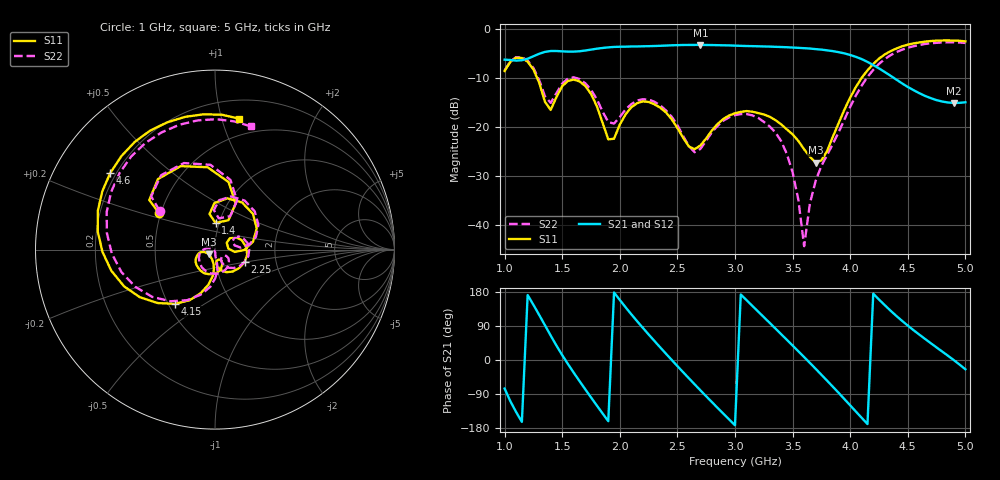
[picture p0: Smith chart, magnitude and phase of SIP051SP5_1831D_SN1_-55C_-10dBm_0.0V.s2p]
# GHz  S  dB  R  50
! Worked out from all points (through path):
!   81 points, 1 GHz to 5 GHz, reference 50 ohm
!   highest |S21| = -3.30 dB at 2.7 GHz (marker M1); lowest = -15.1 dB at 4.9 GHz (marker M2)
!   lowest |S11| = -27.3 dB at 3.7 GHz (marker M3), VSWR 1.09, Z = 46.5 - j2.31 ohm
!   |S11| at or under -10 dB: 1.281 GHz to 4.1 GHz (2.819 GHz wide, 105 % of centre)
!   |S22| runs from -44.3 to -2.8 dB; largest |S21 - S12| = 0.0027
!   S11 on the Smith chart (normalised r, x): 1 GHz: 0.49, +0.23; 1.4 GHz: 0.96, +0.29; 2.25 GHz: 1.38, -0.20; 4.15 GHz: 0.54, -0.38; 4.6 GHz: 0.18, +0.32; 5 GHz: 0.35, +1.14
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1  -8.63 147.1  -6.31 -75.4  -6.31 -75.3  -8.48 144.9
1.2  -6.73 95.1  -6.13 171.4  -6.13 171.4  -6.50 93.1
1.4  -16.57 88.7  -4.55 64.5  -4.56 64.4  -15.12 83.1
1.55  -10.64 76.5  -4.68 -10.8  -4.68 -10.7  -10.17 73.0
1.7  -11.67 27.0  -4.46 -77.3  -4.47 -77.3  -11.12 29.6
1.95  -22.42 30.2  -3.72 178.1  -3.74 178.2  -19.34 25.4
2.1  -16.01 19.3  -3.63 120.6  -3.64 120.6  -15.38 21.1
2.25  -14.94 -23.1  -3.57 67.4  -3.57 67.4  -14.45 -11.0
2.35  -16.08 -51.2  -3.49 33.5  -3.48 33.5  -15.62 -33.5
2.5  -20.24 -82.4  -3.37 -16.1  -3.36 -16.0  -19.66 -59.8
2.7  -23.79 -61.1  -3.30 -80.1  -3.31 -80.1  -24.49 -33.5
3  -17.24 -96.3  -3.46 -172.2  -3.47 -172.2  -17.61 -73.9
3.35  -18.63 -155.3  -3.70 83.3  -3.70 83.3  -21.11 -165.5
3.5  -21.53 -169.7  -3.85 38.1  -3.85 38.1  -29.25 165.1
3.6  -24.58 -166.5  -3.98 7.7  -3.99 7.7  -44.32 -137.0
3.7  -27.30 -145.0  -4.17 -23.1  -4.17 -23.2  -31.01 -85.7
3.9  -19.22 -93.1  -4.79 -86.8  -4.79 -86.8  -21.09 -81.8
4.15  -8.49 -126.5  -6.77 -169.0  -6.77 -169.0  -9.85 -118.8
4.35  -4.59 -168.5  -9.59 130.2  -9.61 130.2  -5.42 -166.5
4.6  -2.82 143.9  -13.15 67.0  -13.16 66.8  -3.33 141.2
4.9  -2.42 94.7  -15.12 -0.4  -15.16 -0.5  -2.77 89.5
5  -2.60 79.5  -15.00 -24.5  -15.00 -24.4  -2.91 73.7
